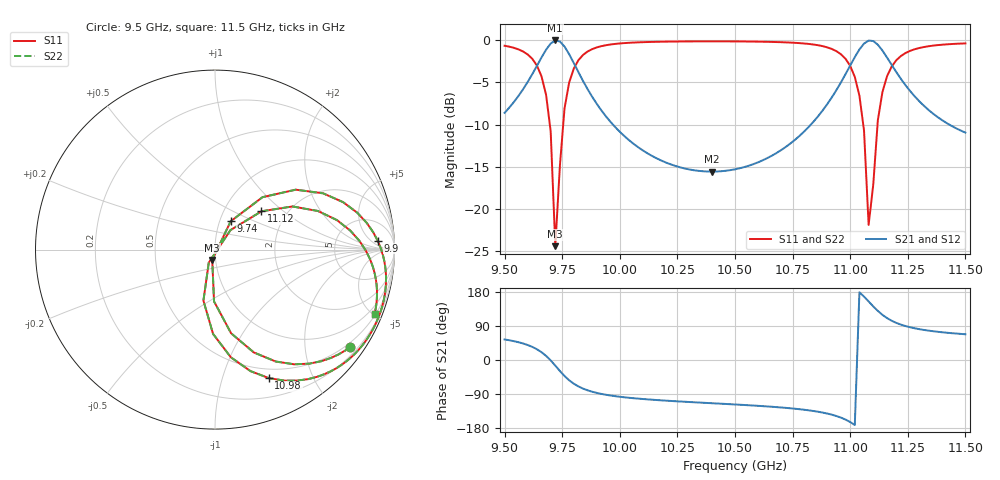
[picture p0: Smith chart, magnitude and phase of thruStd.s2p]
# GHZ S RI R 50
!Output file by EM3DS 6.2.15 Beta
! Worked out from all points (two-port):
!   101 points, 9.5 GHz to 11.5 GHz, reference 50 ohm
!   highest |S21| = -0.02 dB at 9.72 GHz (marker M1); lowest = -15.6 dB at 10.4 GHz (marker M2)
!   |S21| within 3 dB of the highest: 9.64 GHz to 9.806 GHz (165.8 MHz wide, 1.7 % of centre); 11 GHz to 11.18 GHz (182.9 MHz wide, 1.65 % of centre)
!   lowest |S11| = -24.4 dB at 9.72 GHz (marker M3), VSWR 1.13, Z = 48.2 - j5.61 ohm
!   |S11| at or under -10 dB: 9.696 GHz to 9.754 GHz (58.04 MHz wide, 0.597 % of centre); 11.06 GHz to 11.12 GHz (62.06 MHz wide, 0.56 % of centre)
!   |S22| runs from -24.4 to -0.1 dB; largest |S21 - S12| = 2.1e-14
!   S11 on the Smith chart (normalised r, x): 9.5 GHz: 0.39, -3.05; 9.74 GHz: 1.13, +0.37; 9.9 GHz: 16, +9; 10.98 GHz: 0.40, -1.43; 11.12 GHz: 1.49, +0.72; 11.5 GHz: 0.56, -5.07
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9.5  0.7529 -0.5434  0.2173 0.3011  0.2173 0.3011  0.7529 -0.5434
9.6  0.5257 -0.6354  0.4358 0.3606  0.4358 0.3606  0.5257 -0.6354
9.66  0.2164 -0.573  0.7395 0.2793  0.7395 0.2793  0.2164 -0.5731
9.7  -0.00539 -0.2885  0.9573 -0.0179  0.9573 -0.0179  -0.00539 -0.2885
9.72  -0.0153 -0.0581  0.9652 -0.2545  0.9652 -0.2545  -0.0153 -0.0581
9.74  0.0875 0.1578  0.8604 -0.4767  0.8604 -0.4767  0.0875 0.1578
9.76  0.2648 0.2921  0.6809 -0.6172  0.6809 -0.6172  0.2648 0.2921
9.78  0.4497 0.3338  0.4938 -0.6652  0.4938 -0.6652  0.4497 0.3338
9.84  0.7914 0.2066  0.1453 -0.5567  0.1453 -0.5567  0.7914 0.2066
9.9  0.9062 0.05  0.0231 -0.4191  0.0231 -0.4191  0.9062 0.0501
10.18  0.9409 -0.278  -0.0548 -0.1856  -0.0548 -0.1856  0.9409 -0.278
10.4  0.9004 -0.4021  -0.0678 -0.1519  -0.0678 -0.1519  0.9004 -0.4021
10.52  0.8692 -0.4628  -0.0818 -0.1536  -0.0818 -0.1536  0.8692 -0.4628
10.84  0.6734 -0.6625  -0.2301 -0.2339  -0.2301 -0.2339  0.6734 -0.6625
10.98  0.2997 -0.7158  -0.5818 -0.2436  -0.5818 -0.2436  0.2997 -0.7158
11.04  -0.0108 -0.4697  -0.8825 0.0204  -0.8825 0.0204  -0.0108 -0.4697
11.06  -0.0645 -0.2843  -0.9329 0.2117  -0.9329 0.2117  -0.0645 -0.2843
11.08  -0.0346 -0.0724  -0.8995 0.4294  -0.8995 0.4294  -0.0346 -0.0724
11.12  0.2591 0.2135  -0.5991 0.7269  -0.5991 0.7269  0.2591 0.2135
11.18  0.6794 0.1644  -0.1682 0.6951  -0.1682 0.6951  0.6794 0.1644
11.28  0.88 -0.0971  0.051 0.4621  0.051 0.4621  0.88 -0.0971
11.5  0.8887 -0.3604  0.1065 0.2626  0.1065 0.2626  0.8887 -0.3604
